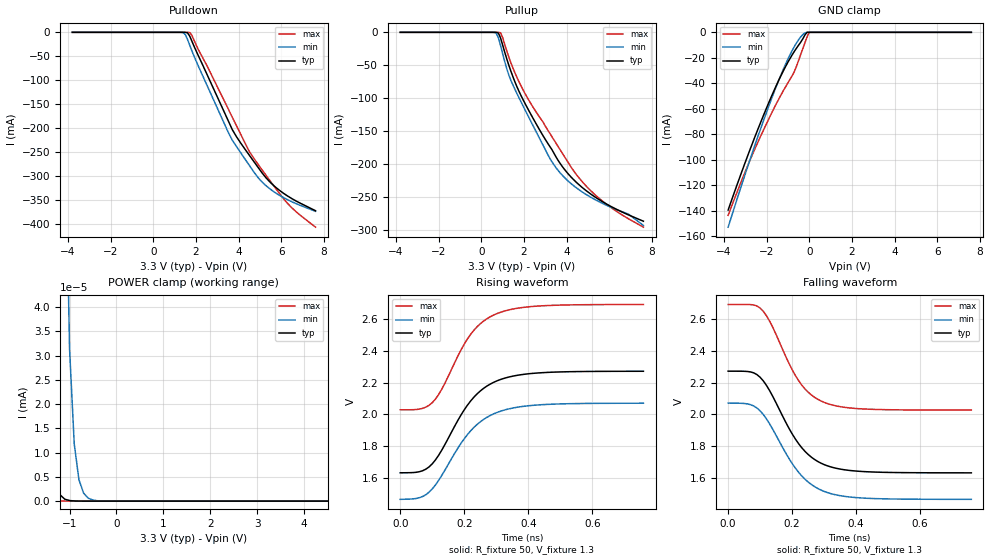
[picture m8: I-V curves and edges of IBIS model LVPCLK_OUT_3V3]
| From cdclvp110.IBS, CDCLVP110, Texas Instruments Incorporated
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|   Diff. Driver Output Model for 3.3V VCC range   |
[Model]   LVPCLK_OUT_3V3
Model_type   3-state_ECL
| Signals   Y0,Y0-, Y1,Y1-, y2,Y2-, y3,y3-, y4,y4-
|   y5,y5-, y6,y6-, y7,y7-, y8,y8-, y9,y9-
| variable   typ   min   max
C_comp   2.5pF   NA   NA
Cref = 0pF   |load capacitance for timing spec
Rref = 50   |50 to VCC-2
Vref = 1.3   |Timing specification test load voltage, VCC-2V
Vmeas = 1.95V   |Vref for timing measurements (x-point)
[Model Spec]
Vmeas   1.95V   1.77V   2.36V
| Vmeas is the expected cross point for each differential signal pair.
|Vref   1.3V   1.0V   1.8V
[Temperature Range]   40C   110C   -40C
[Voltage range]   3.3V   3.0V   3.8V
[Pulldown reference]   3.3V   3.0V   3.8V
[GND Clamp reference]   0V   0V   0V
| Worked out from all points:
|   GND clamp passes 1 mA (typ) near -0.15 V on its own axis
|   POWER clamp passes 1 mA (typ) near -2.34 V on its own axis
|   rising waveform, R_fixture 50, V_fixture 1.3: 20-80 % time 123ps typ, 127ps min, 114ps max; typ from 1.63 V to 2.27 V
|   falling waveform, R_fixture 50, V_fixture 1.3: 20-80 % time 113ps typ, 117ps min, 104ps max; typ from 2.27 V to 1.63 V
[Pullup]
|   40C:3.3V:nominal   110C:3.0V:weak   -40C:3.8:strong
|  Voltage   I(typ)   I(min)   I(max)
-3.8V     62.91pA    249.9pA    61.33pA
600mV     -1.193uA   -94.4uA    -441.6pA
700mV     -41.8uA    -1.388mA   -54.72nA
900mV     -8.202mA   -19.73mA   -667.2uA
1.3V      -50.76mA   -65.61mA   -38.39mA
1.8V      -91.65mA   -101.2mA   -77.11mA
3.2V      -172.3mA   -190.2mA   -152.4mA
3.6V      -193.9mA   -209.2mA   -172.9mA
4.5V      -228.6mA   -236.6mA   -217.2mA
5.3V      -248.8mA   -252.9mA   -245.2mA
6.9V      -276.6mA   -275.5mA   -282.4mA
7.6V      -286.2mA   -292.6mA   -295.2mA
[Pulldown]
|   40C:3.3V:nominal   110C:3.0V:weak   -40C:3.8:strong
|  Voltage   I(typ)   I(min)   I(max)
-3.8V     70.21pA    262.9pA    68.55pA
1.3V      -54.47nA   -47.49uA   -18.68pA
1.5V      -48.29uA   -5.059mA   -38.51nA
1.7V      -7.636mA   -26.4mA    -356.3uA
2.1V      -48.12mA   -69.81mA   -35.46mA
3.7V      -203.3mA   -225.5mA   -177.3mA
4.5V      -256.8mA   -278mA     -249.2mA
4.9V      -281.5mA   -303mA     -275.1mA
5.3V      -304.8mA   -321mA     -299.8mA
5.9V      -329.7mA   -340.1mA   -336mA
6.5V      -347.6mA   -354mA     -366.9mA
7.6V      -372.6mA   -373.9mA   -406.9mA
[POWER Clamp]
|   40C:3.3V:nominal   110C:3.0V:weak   -40C:3.8:strong
|  Voltage   I(typ)   I(min)   I(max)
-3.9V     57.26mA    62.57mA    49.46mA
-2.1V     57.9uA     1.163mA    92.06nA
-1.9V     5.436uA    193.3uA    3.702nA
-1.7V     502nA      28.57uA    168.1pA
-1.5V     46.03nA    4.117uA    22.74pA
-1.4V     13.92nA    1.558uA    15.79pA
-1.3V     4.21nA     588.3nA    12.73pA
-1.1V     390.6pA    83.61nA    8.748pA
-1V       122.4pA    31.45nA    7.116pA
-900mV    40.5pA     11.81nA    5.657pA
-600mV    3.301pA    602.5pA    2.284pA
7.6V      0A         0A         0A
[GND Clamp]
|   40C:3.3V:nominal   110C:3.0V:weak   -40C:3.8:strong
|  Voltage   I(typ)   I(min)   I(max)
-3.8V     -139.3mA   -152.7mA   -143.4mA
-3.2V     -111.1mA   -121.3mA   -117.5mA
-2.6V     -84.28mA   -91.1mA    -93.39mA
-2V       -59.3mA    -62.65mA   -71.59mA
-1.6V     -43.78mA   -44.81mA   -57.86mA
-1.2V     -29.75mA   -28.44mA   -45.37mA
-700mV    -15.03mA   -11.24mA   -30.85mA
-500mV    -10.13mA   -5.863mA   -22.12mA
-300mV    -5.129mA   -1.783mA   -12.8mA
-100mV    0A         0A         -3.549mA
0V        0A         0A         0A
7.6V      0A         0A         0A
[ramp]
| variable   typ   min   max
dV/dt_r   0.4062/1.3364E-10   0.3779/1.3504E-10   0.4103/1.1853E-10
dV/dt_f   0.4062/1.2047E-10   0.3779/1.2198E-10   0.4103/1.0706E-10
[Rising Waveform]
R_fixture = 50
V_fixture = 1.3
V_fixture_min = 1.0
V_fixture_max = 1.8
|   40C:3.3V:nominal  110C:3.0V:weak -40C:3.8:strong
|  Voltage   V(typ)   V(min)   V(max)
0s        1.631V     1.464V     2.028V
60ps      1.638V     1.474V     2.033V
100ps     1.687V     1.529V     2.073V
130ps     1.775V     1.615V     2.159V
190ps     1.996V     1.817V     2.406V
220ps     2.084V     1.896V     2.505V
260ps     2.163V     1.967V     2.588V
300ps     2.209V     2.01V      2.634V
430ps     2.261V     2.059V     2.683V
760ps     2.272V     2.07V      2.693V
[Falling Waveform]
R_fixture = 50
V_fixture = 1.3
V_fixture_min = 1.0
V_fixture_max = 1.8
|   40C:3.3V:nominal  110C:3.0V:weak -40C:3.8:strong
|  Voltage   V(typ)   V(min)   V(max)
0s        2.272V     2.071V     2.693V
70ps      2.268V     2.061V     2.692V
100ps     2.234V     2.022V     2.671V
130ps     2.148V     1.938V     2.587V
190ps     1.912V     1.722V     2.322V
220ps     1.815V     1.635V     2.213V
260ps     1.73V      1.557V     2.122V
300ps     1.683V     1.514V     2.076V
420ps     1.639V     1.472V     2.034V
760ps     1.631V     1.464V     2.027V
